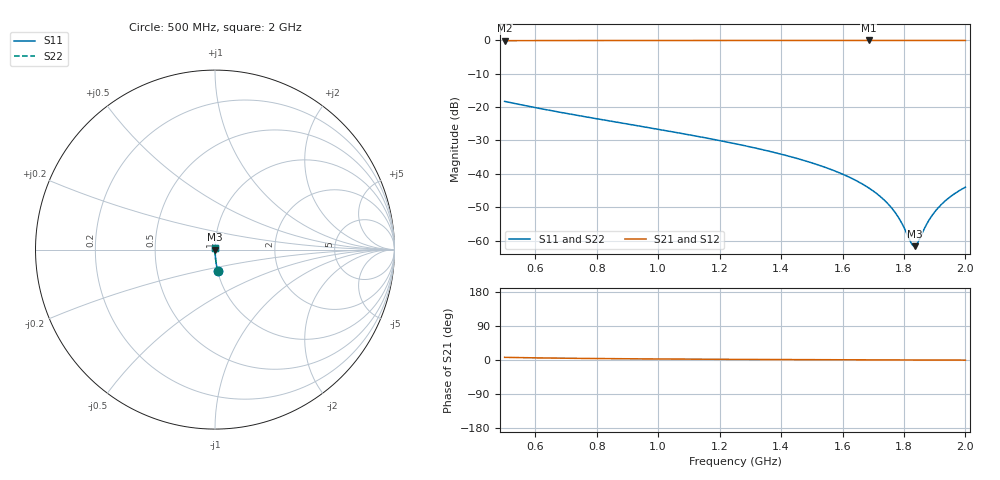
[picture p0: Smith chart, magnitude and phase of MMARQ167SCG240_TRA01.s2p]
! MMARQ167SCG240_TRA01  S-PARAMETER MODEL  ( General Type )
! Model Generated by TAIYO YUDEN Corporation (http://www.ty-top.com)
! Version 1.0
! TAIYO YUDEN Control No. 160201
! Copyright(c) 2016 TAIYO YUDEN CO.,LTD. All Rights Reserved.
! Product Description (link to TY-COMPAS)
! https://ds.yuden.co.jp/TYCOMPAS/or/detail?pn=MMARQ167SCG240JTRA01&u=M
! Products Name : Multilayer Ceramic Capacitors
! Characteristics :
!  Capacitance : 24 pF , Rated Voltage : 250V , TCC : CG / C0G
!  Case Size : 1.6 x 0.8 / 0.063 x 0.031 [mm/inch] , Thickness : 0.7 / 0.028 [mm/inch]
!  (Conditions: Temperature = 25 degC , DC Bias Current/Voltage = 0A / 0V)
! External Node Assignments :
!  1  o---| |---o  2
! GND o---------o GND
! Frequency Range : 500MHz  -  2000MHz  [ 401 STEP ]
# MHz S RI R 50
! Freq[MHz].  S11 Real  S11 Imag  S21 Real  S21 Imag  S12 Real  S12 Imag  S22 Real  S22 Imag
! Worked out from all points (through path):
!   401 points, 500 MHz to 2 GHz, reference 50 ohm
!   highest |S21| = -0.01 dB at 1.685 GHz (marker M1); lowest = -0.1 dB at 500 MHz (marker M2)
!   group delay of S21, straight-line fit = 11.9 ps
!   lowest |S11| = -61.7 dB at 1.835 GHz (marker M3), VSWR 1.00, Z = 50.1 + j0.00392 ohm
!   |S11| at or under -10 dB: start of sweep to end of sweep
!   |S22| runs from -61.7 to -18.3 dB; largest |S21 - S12| = 0
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500  0.0153 -0.1211  0.9847 0.1211  0.9847 0.1211  0.0153 -0.1211
751.25  0.00584 -0.073  0.9942 0.073  0.9942 0.073  0.00584 -0.073
1002.5  0.00271 -0.0462  0.9973 0.0462  0.9973 0.0462  0.00271 -0.0462
1250  0.00146 -0.0283  0.9985 0.0283  0.9985 0.0283  0.00146 -0.0283
1388.75  0.00111 -0.0203  0.9989 0.0203  0.9989 0.0203  0.00111 -0.0203
1501.25  0.000944 -0.0145  0.9991 0.0145  0.9991 0.0145  0.000944 -0.0145
1606.25  0.000854 -0.00958  0.9991 0.00958  0.9991 0.00958  0.000854 -0.00958
1685  0.000821 -0.00611  0.9992 0.00611  0.9992 0.00611  0.000821 -0.00611
1722.5  0.000814 -0.00452  0.9992 0.00452  0.9992 0.00452  0.000814 -0.00452
1752.5  0.000812 -0.00327  0.9992 0.00327  0.9992 0.00327  0.000812 -0.00327
1771.25  0.000812 -0.00251  0.9992 0.00251  0.9992 0.00251  0.000812 -0.00251
1786.25  0.000813 -0.0019  0.9992 0.0019  0.9992 0.0019  0.000813 -0.0019
1823.75  0.000819 -0.000404  0.9992 0.000404  0.9992 0.000404  0.000819 -0.000404
1831.25  0.000821 -0.000108  0.9992 0.000108  0.9992 0.000108  0.000821 -0.000108
1835  0.000822 3.91e-05  0.9992 -3.91e-05  0.9992 -3.91e-05  0.000822 3.91e-05
1838.75  0.000823 0.000186  0.9992 -0.000186  0.9992 -0.000186  0.000823 0.000186
1846.25  0.000825 0.000479  0.9992 -0.000479  0.9992 -0.000479  0.000825 0.000479
1868.75  0.000832 0.00135  0.9992 -0.00135  0.9992 -0.00135  0.000832 0.00135
1883.75  0.000838 0.00193  0.9992 -0.00193  0.9992 -0.00193  0.000838 0.00193
1910  0.000849 0.00292  0.9992 -0.00292  0.9992 -0.00292  0.000849 0.00292
1951.25  0.00087 0.00446  0.9991 -0.00446  0.9991 -0.00446  0.00087 0.00446
2000  0.000901 0.00624  0.9991 -0.00624  0.9991 -0.00624  0.000901 0.00624
